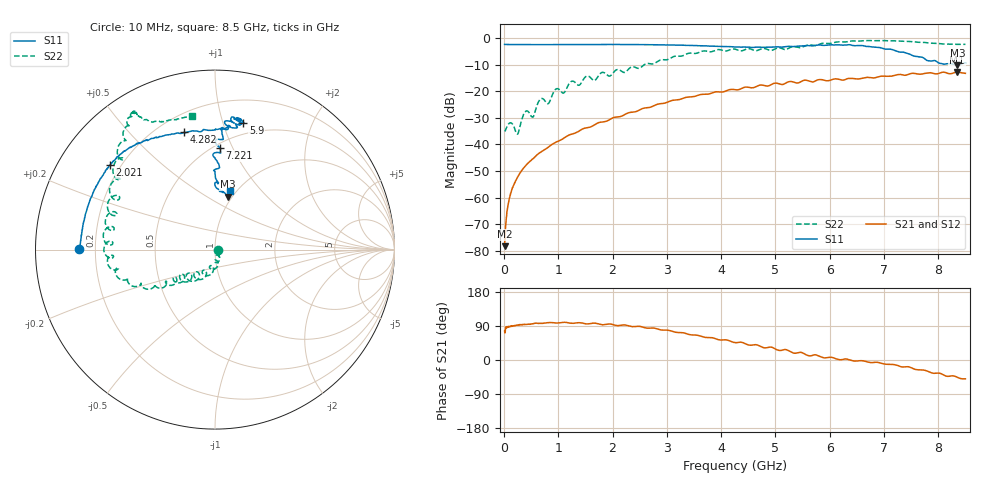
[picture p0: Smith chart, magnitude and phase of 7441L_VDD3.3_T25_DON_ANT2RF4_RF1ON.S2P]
!Agilent Technologies,E5071C,MY46417908,A.11.23
!Date: Mon May 03 19:53:47 2021
!Data & Calibration Information:
!Freq	S11:SOLT2(ON)	S21:SOLT2(ON)	S12:SOLT2(ON)	S22:SOLT2(ON)
!PortZ  Port1:50+j0  Port2:50+j0
!Above PortZ is port z conversion or system Z0 setting when saving the data.
!When reading, reference impedance value at option line is always used.
# Hz S dB R 50
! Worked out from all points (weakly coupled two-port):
!   1601 points, 10 MHz to 8.5 GHz, reference 50 ohm
!   highest |S21| = -12.84 dB at 8.346 GHz (marker M1); lowest = -78.3 dB at 10 MHz (marker M2)
!   lowest |S11| = -10.4 dB at 8.351 GHz (marker M3), VSWR 1.87, Z = 47.9 + j31.1 ohm
!   |S11| at or under -10 dB: 8.293 GHz to 8.415 GHz (122.3 MHz wide, 1.46 % of centre)
!   |S22| runs from -36.2 to -1.0 dB; largest |S21 - S12| = 0.0016
!   S11 on the Smith chart (normalised r, x): 10 MHz: 0.14, +0.00; 2.021 GHz: 0.16, +0.34; 4.282 GHz: 0.30, +0.73; 5.9 GHz: 0.40, +1.17; 7.221 GHz: 0.53, +0.89; 8.5 GHz: 0.94, +0.70
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1e7  -2.44 179.7  -78.27 76.1  -78.41 73.1  -35.15 -0.8
6.836875e7  -2.48 178.5  -63.39 87.8  -63.13 86.2  -32.84 -14.3
1.16125e8  -2.48 177.5  -59.00 89.2  -58.90 89.2  -31.88 -34.3
2.43475e8  -2.51 174.8  -52.56 92.2  -52.49 91.7  -36.17 -49.7
3.336812e8  -2.52 172.9  -49.57 93.7  -49.57 93.7  -30.13 -39.3
4.079688e8  -2.53 171.3  -47.81 93.9  -47.78 93.6  -27.45 -64.3
5.353188e8  -2.52 168.6  -45.37 96.0  -45.31 95.8  -29.65 -67.9
6.785875e8  -2.53 165.5  -42.90 96.7  -42.91 96.7  -22.85 -78.5
8.218562e8  -2.53 162.8  -40.94 98.9  -40.94 99.0  -24.56 -84.1
9.598188e8  -2.51 160.0  -39.15 97.7  -39.16 97.6  -19.16 -93.6
1.426769e9  -2.50 151.6  -34.45 98.0  -34.44 98.0  -16.79 -109.2
2.021069e9  -2.49 141.3  -29.92 92.7  -29.92 92.8  -12.85 -129.5
2.843538e9  -2.59 130.4  -24.85 81.0  -24.86 81.1  -8.63 -144.6
4.255e9  -3.43 105.5  -19.46 45.9  -19.46 45.9  -4.23 177.8
4.281531e9  -3.41 104.7  -19.53 45.7  -19.54 45.6  -4.37 176.2
5.671769e9  -2.97 78.4  -16.54 11.6  -16.49 11.6  -2.72 135.6
5.899938e9  -2.82 77.4  -15.93 5.5  -15.88 5.7  -2.02 130.8
7.088538e9  -4.22 88.1  -14.40 -11.5  -14.44 -11.5  -1.10 120.3
7.221194e9  -4.91 87.3  -13.94 -13.3  -13.95 -13.4  -1.09 120.0
8.346119e9  -10.35 76.4  -12.84 -45.4  -12.87 -45.5  -2.41 104.9
8.351425e9  -10.36 76.3  -12.84 -45.7  -12.88 -45.9  -2.42 104.7
8.5e9  -9.39 75.4  -13.32 -49.7  -13.35 -49.8  -2.42 99.8
